PROGRAM MAIN
VAR
	wArrScannerFromAdapter_1			AT%I*		:ARRAY[0..247] OF WORD;
	wArrScannerToAdapter_1				AT%Q*		:ARRAY[0..247] OF WORD;
	wArrScannerFromAdapter_2			AT%I*		:ARRAY[0..247] OF WORD;
	wArrScannerToAdapter_2				AT%Q*		:ARRAY[0..247] OF WORD;
	wArrScannerFromAdapter_3			AT%I*		:ARRAY[0..247] OF WORD;
	wArrScannerToAdapter_3				AT%Q*		:ARRAY[0..247] OF WORD;
	wArrScannerFromAdapter_4			AT%I*		:ARRAY[0..247] OF WORD;
	wArrScannerToAdapter_4				AT%Q*		:ARRAY[0..247] OF WORD;
	wArrScannerFromAdapter_5			AT%I*		:ARRAY[0..247] OF WORD;
	wArrScannerToAdapter_5				AT%Q*		:ARRAY[0..247] OF WORD;
	wArrScannerFromAdapter_6			AT%I*		:ARRAY[0..247] OF WORD;
	wArrScannerToAdapter_6				AT%Q*		:ARRAY[0..247] OF WORD;
	wArrScannerFromAdapter_7			AT%I*		:ARRAY[0..247] OF WORD;
	wArrScannerToAdapter_7				AT%Q*		:ARRAY[0..247] OF WORD;
	wArrScannerFromAdapter_8			AT%I*		:ARRAY[0..247] OF WORD;
	wArrScannerToAdapter_8				AT%Q*		:ARRAY[0..247] OF WORD;
	i,j												:INT;
	
END_VAR

FOR i:=0 TO 247 DO
	wArrScannerToAdapter_1[i]				:=i+1;
END_FOR


FOR j:=0 TO 247 DO
	wArrScannerToAdapter_8[j]				:=j+1;
END_FOR

END_PROGRAM
